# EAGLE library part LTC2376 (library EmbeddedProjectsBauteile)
LTC2376-16 - 16-Bit, 250ksps, Low Power SAR ADC with 97dB SNR
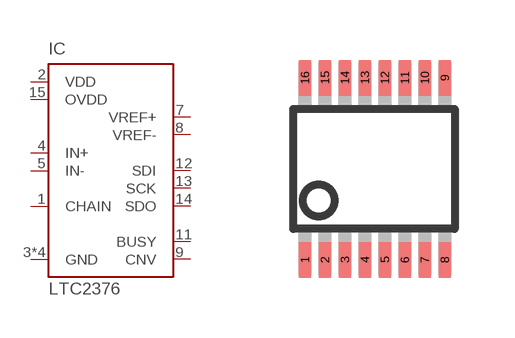
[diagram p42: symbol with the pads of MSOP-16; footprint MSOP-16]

Designator prefix IC

## LTC2376 (EP: 401441)  [MSOP-16]
1  CHAIN  in
2  VDD  pwr
3  GND  pwr
4  IN+  in
5  IN-  in
6  GND  pwr
7  VREF+  in
8  VREF-  in
9  CNV  in
10  GND  pwr
11  BUSY  out
12  SDI  in
13  SCK  in
14  SDO  out
15  OVDD  pwr
16  GND  pwr

## Footprint MSOP-16 (pad centres in mm)
smd 0.305 x 0.889: 1 -1.725,-2.275; 2 -1.225,-2.275; 3 -0.725,-2.275; 4 -0.225,-2.275; 5 0.275,-2.275; 6 0.775,-2.275; 7 1.275,-2.275; 8 1.775,-2.275; 9 1.775,2.275; 10 1.275,2.275; 11 0.775,2.275; 12 0.275,2.275; 13 -0.225,2.275; 14 -0.725,2.275; 15 -1.225,2.275; 16 -1.725,2.275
